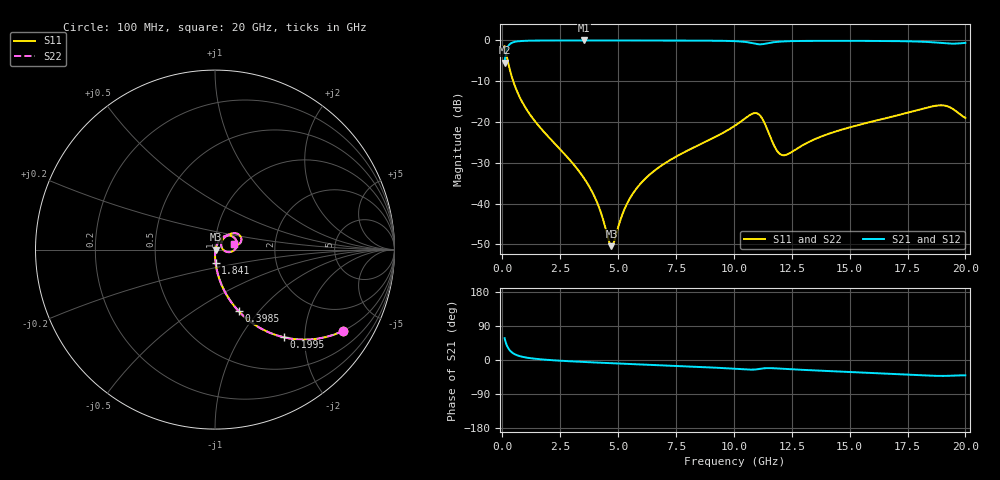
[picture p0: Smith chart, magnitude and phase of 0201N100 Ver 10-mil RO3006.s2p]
# GHz S MA R 50
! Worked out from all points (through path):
!   1601 points, 100 MHz to 20 GHz, reference 50 ohm
!   highest |S21| = -0.02 dB at 3.52 GHz (marker M1); lowest = -5.5 dB at 100 MHz (marker M2)
!   group delay of S21, straight-line fit = 7.19 ps
!   lowest |S11| = -50.4 dB at 4.714 GHz (marker M3), VSWR 1.01, Z = 50.3 - j0.0581 ohm
!   |S11| at or under -10 dB: 471 MHz to end of sweep
!   |S22| runs from -50.4 to -1.5 dB; largest |S21 - S12| = 0
!   S11 on the Smith chart (normalised r, x): 100 MHz: 0.99, -3.16; 199.5 MHz: 0.99, -1.58; 398.5 MHz: 0.99, -0.79; 1.841 GHz: 1.00, -0.15; 20 GHz: 1.24, +0.07
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0.1  0.8456 -32.4  0.5331 57.6  0.5331 57.6  0.8456 -32.4
0.1995  0.6214 -51.9  0.7826 38.1  0.7826 38.1  0.6214 -51.9
0.2865625  0.4827 -61.5  0.8748 28.3  0.8748 28.3  0.4827 -61.5
0.3985  0.3674 -69.0  0.929 20.8  0.929 20.8  0.3674 -69.0
0.94575  0.1591 -82.1  0.9859 7.4  0.9859 7.4  0.1591 -82.1
1.84125  0.07328 -87.7  0.9954 0.9  0.9954 0.9  0.07328 -87.7
3.420812  0.02268 -88.5  0.9971 -4.9  0.9971 -4.9  0.02268 -88.5
3.520313  0.02067 -88.1  0.9971 -5.2  0.9971 -5.2  0.02067 -88.1
4.092437  0.01037 -81.3  0.9971 -6.8  0.9971 -6.8  0.01037 -81.3
4.714313  0.003011 -11.1  0.9969 -8.5  0.9969 -8.5  0.003011 -11.1
5.236688  0.008031 56.6  0.9966 -9.9  0.9966 -9.9  0.008031 56.6
5.560062  0.01224 63.5  0.9965 -10.7  0.9965 -10.7  0.01224 63.5
6.741625  0.02753 68.2  0.9956 -13.7  0.9956 -13.7  0.02753 68.2
10.05  0.09018 55.2  0.9775 -23.1  0.9775 -23.1  0.09018 55.2
11.045  0.126 13.5  0.8971 -24.2  0.8971 -24.2  0.126 13.5
11.28131  0.103 -3.5  0.9016 -22.1  0.9016 -22.1  0.103 -3.5
11.81612  0.04665 -2.2  0.9557 -22.0  0.9557 -22.0  0.04665 -2.2
12.10219  0.03923 17.1  0.9694 -23.1  0.9694 -23.1  0.03923 17.1
13.37081  0.05932 50.4  0.9852 -27.2  0.9852 -27.2  0.05932 50.4
16.69162  0.1136 47.7  0.9809 -36.1  0.9809 -36.1  0.1136 47.7
18.94281  0.1601 26.2  0.9289 -42.0  0.9289 -42.0  0.1601 26.2
20  0.1121 14.8  0.9315 -40.6  0.9315 -40.6  0.1121 14.8
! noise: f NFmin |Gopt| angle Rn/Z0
0.1  0.0007127  0.9397  0.3571  0.002638
2.301  0.004312  0.788  4.241  0.004183
4.515  0.007224  0.7565  8.146  0.00597
6.729  0.01017  0.7447  12.04  0.007915
8.943  0.01574  0.7774  15.94  0.01419
11.14  0.07032  0.9328  19.94  0.2257
13.36  0.02584  0.7971  23.75  0.02525
15.57  0.02491  0.7609  27.48  0.01995
17.79  0.03763  0.8149  31.33  0.03941
20  0.0715  0.8869  35.22  0.1248
